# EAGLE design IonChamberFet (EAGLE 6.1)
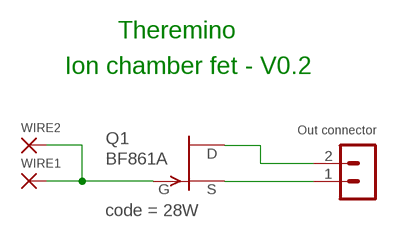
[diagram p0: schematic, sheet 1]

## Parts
OUT  Out connector  MA02-1L2  [MA02-1_L2]
Q1  BF861A  BF861L  [SOT23_L]
WIRE1  WIREPAD1,6/0,8  [1,6/0,8]
WIRE2  WIREPAD1,6/0,8  [1,6/0,8]

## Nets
DRAIN: OUT.2 Q1.1(D)
GATE: Q1.3(G) WIRE1.1(P) WIRE2.1(P)
GND: OUT.1 Q1.2(S)

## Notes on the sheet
- Theremino
- Ion chamber fet - V0.2

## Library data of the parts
OUT = 03-con-lstb-M:MA02-1: PIN HEADER
Q1 = 00-LIVIO:BF861; MARKCODE: code = 28W
WIRE1 WIRE2 = 00-LIVIO:WIREPAD: Wire PAD connect wire on PCB

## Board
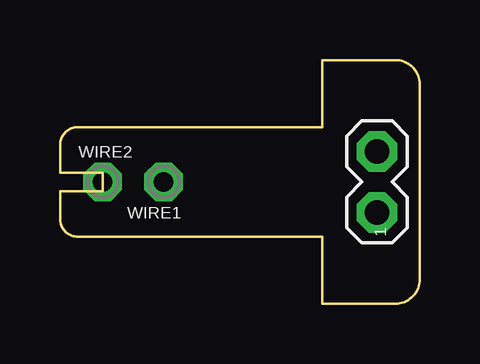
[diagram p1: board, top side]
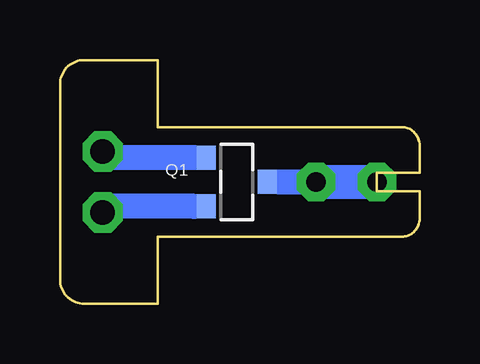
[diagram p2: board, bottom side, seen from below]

Size 14.99 x 10.16 mm. Coordinates in mm from the lower left corner, seen from the top.
Outline: 0,3.56 arc90 0.76,2.79 10.92,2.79 10.92,0 13.97,0 arc90 14.99,1.02 14.99,9.14 arc90 13.97,10.16 10.92,10.16 10.92,7.37 0.76,7.37 arc90 0,6.6 0,5.46 1.78,5.46 1.78,4.7 0,4.7 0,3.56
Copper layers (1*16): Top 0.035mm / dielectric 1.5mm / Bottom 0.035mm
Design rules: minimum track width 10mil, minimum drill 27mil, track to track 27mil, track to pad 27mil, pad to pad 27mil, via to via 27mil, smd to smd 27mil, copper to edge 27mil, drill to drill 8mil, minimum pad ring 5mil, minimum via ring 8mil, stop-mask expansion 4mil, vias tented up to drill 0mil, thermal gap 41mil

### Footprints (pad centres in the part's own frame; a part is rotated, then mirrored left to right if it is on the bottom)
MA02-1_L2 = drill 1.016 pad 1.676 octagon: 1 -1.27,0; 2 1.27,0
SOT23_L = smd 1 x 0.8: 1 -1.016,-1.27; 2 1.016,-1.27; 3 0,1.27
1,6/0,8 = drill 0.813 pad 1.6 octagon: 1 0,0

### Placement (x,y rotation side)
OUT  13.21,5.08 90 top
Q1  7.62,5.08 270 bottom
WIRE1  4.32,5.08 0 top
WIRE2  1.78,5.08 0 top

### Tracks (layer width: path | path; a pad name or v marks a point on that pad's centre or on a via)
DRAIN
  Bottom 0.813: Q1.1 9.4,6.1
  Bottom 1.05: 9.4,6.1 12.95,6.1 OUT.2
GATE
  Bottom 0.813: Q1.3 5.84,5.08
  Bottom 1.05: 5.84,5.08 WIRE1.1
  Bottom 1.422: WIRE1.1 WIRE2.1
GND
  Bottom 0.813: Q1.2 9.4,4.06
  Bottom 1.05: 9.4,4.06 12.95,4.06 OUT.1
